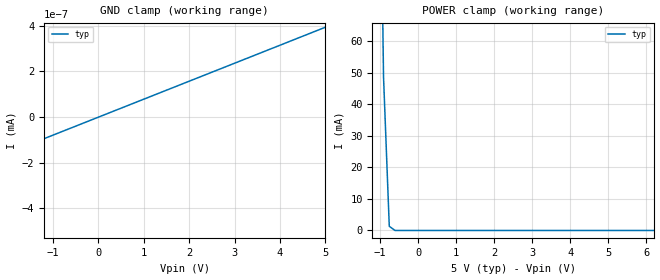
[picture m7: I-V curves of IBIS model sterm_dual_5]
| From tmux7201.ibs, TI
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| sterm_dual_5
[Model]   sterm_dual_5
Model_type   Terminator
|   typ   min   max
C_comp   2.533030e-11   NA   NA
[Voltage Range]   5   NA   NA
[Temperature Range]   27   NA   NA
[Power Clamp Reference]   5   NA   NA
[GND Clamp Reference]   0   NA   NA
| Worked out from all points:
|   GND clamp passes 1 mA (typ) near -5.72 V on its own axis
|   POWER clamp passes 1 mA (typ) near -0.72 V on its own axis
[GND Clamp]
|   Voltage   I(typ)   I(min)   I(max)
-10V      -9.854A    NA         NA
-5.303V   -789.5pA   NA         NA
-5.152V   -411pA     NA         NA
-5V       -394.1pA   NA         NA
5V        393.6pA    NA         NA
[POWER Clamp]
|   Voltage   I(typ)   I(min)   I(max)
-5V       13.26A     NA         NA
-1.061V   184.1mA    NA         NA
-909.1mV  48.7mA     NA         NA
-757.6mV  1.324mA    NA         NA
-606.1mV  6.572uA    NA         NA
10V       -394.1pA   NA         NA
